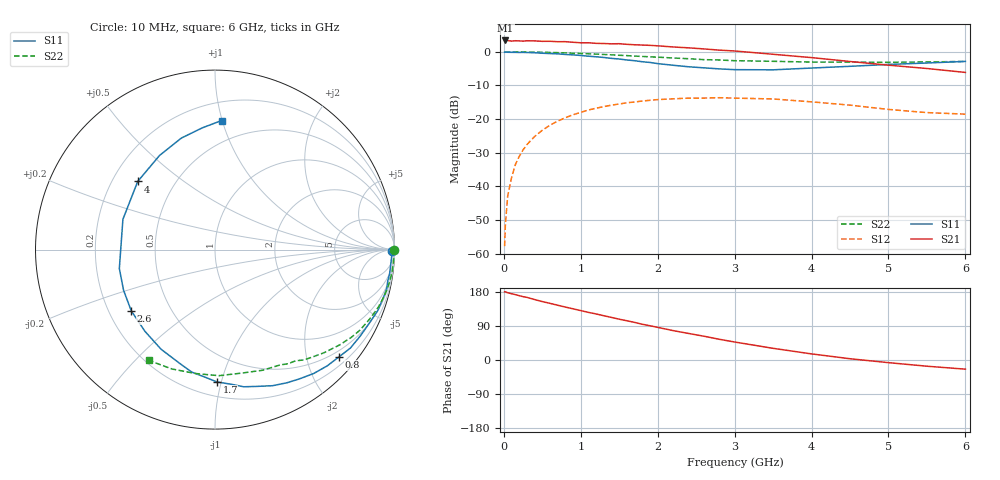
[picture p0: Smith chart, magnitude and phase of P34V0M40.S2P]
! SIEMENS Small Signal Semiconductors
! BFP181
! Si NPN RF Bipolar Junction Transistor in SOT143
! VCE = 4 V  IC = 0.4 mA
! Common Emitter S-Parameters:  March  1996
# GHz  S  MA  R  50
!  f  S11  S21  S12  S22
! GHz  MAG  ANG  MAG  ANG  MAG  ANG  MAG  ANG
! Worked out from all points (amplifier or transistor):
!   36 points, 10 MHz to 6 GHz, reference 50 ohm
!   highest |S21| = 3.4 dB at 20 MHz (marker M1)
!   |S21| within 3 dB of that: start of sweep to 2.903 GHz
!   unconditionally stable (mu >= 1): 3.89 GHz to end of sweep
!   at 250 MHz: K = 0.08, MSG = 16.1 dB, |S12| = -29.1 dB
!   at 1.4 GHz: K = 0.42, MSG = 9.1 dB, |S12| = -15.8 dB
!   at 6 GHz: K = 1.50, MAG = 2.0 dB, |S12| = -18.5 dB
!   S11 on the Smith chart (normalised r, x): 10 MHz: open; 800 MHz: 0.37, -2.64; 1.7 GHz: 0.30, -0.97; 2.6 GHz: 0.29, -0.30; 4 GHz: 0.31, +0.35; 6 GHz: 0.33, +0.99
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0.01  0.9865 -0.6  1.452 179.9  0.0013 91.6  0.9992 -0.2
0.02  0.9915 -1.1  1.474 179.7  0.0027 94.4  0.9972 -0.5
0.05  0.9852 -2.2  1.469 177.5  0.0072 89.8  0.9974 -1.3
0.1  0.9824 -5.2  1.442 174.9  0.0135 84.7  0.9977 -2.5
0.15  0.9821 -7.8  1.46 172.5  0.0212 83.7  0.9964 -3.8
0.2  0.9783 -10.2  1.451 169.8  0.028 82.6  0.9963 -5.0
0.3  0.9763 -15.4  1.459 165.3  0.0419 78.8  0.9934 -7.6
0.4  0.9689 -20.4  1.452 159.5  0.0552 75.0  0.9897 -10.1
0.6  0.9418 -30.7  1.433 149.5  0.0814 67.6  0.9787 -15.0
0.8  0.9132 -40.9  1.414 139.7  0.1051 60.3  0.9636 -19.7
1.1  0.8605 -56.8  1.361 125.6  0.1367 49.8  0.9333 -26.6
1.5  0.7808 -78.2  1.319 107.7  0.168 36.9  0.8877 -35.0
1.7  0.7372 -89.2  1.272 99.2  0.1799 31.0  0.8637 -38.9
1.9  0.6948 -100.7  1.247 90.4  0.1904 25.3  0.8423 -42.4
2.2  0.6313 -118.4  1.18 77.6  0.2003 17.4  0.8091 -47.6
2.6  0.578 -143.8  1.104 62.8  0.2055 8.0  0.7649 -54.1
3  0.5433 -168.8  1.029 47.5  0.2052 -1.4  0.7378 -60.6
3.5  0.5401 161.8  0.919 30.8  0.1994 -10.8  0.7225 -68.5
4  0.5741 138.6  0.82 16.1  0.1807 -18.3  0.7039 -77.9
4.5  0.6088 120.5  0.718 3.3  0.1615 -24.1  0.7028 -88.2
5.5  0.6818 96.0  0.565 -16.4  0.1251 -22.0  0.7069 -109.7
6  0.72 87.1  0.494 -24.2  0.1187 -17.4  0.7194 -120.9
